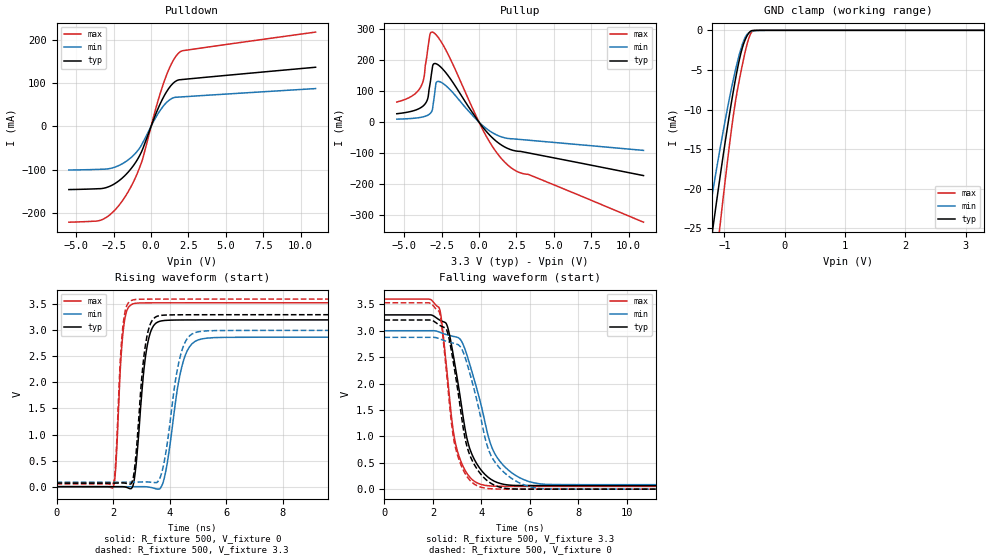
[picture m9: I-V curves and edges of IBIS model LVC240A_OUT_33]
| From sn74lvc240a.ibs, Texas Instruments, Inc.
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[Model]   LVC240A_OUT_33
Model_type  3-state
Enable   Active-Low
Vref =   0
Rref =   500
Cref =   50p
Vmeas =   1.5
| variable   typ   min   max
C_comp   5.30pF   4.90pF   6.71pF
| C_pullup   7.07pF   5.60pF   8.53pF
| C_pulldown   6.30pF   4.97pF   7.29pF
| C_tri-state   5.30pF   4.90pF   6.71pF
[Temperature Range]   40   100   -40
| Ambient temperature   25   85   -40
[Voltage range]   3.3   3   3.6
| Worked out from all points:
|   slope of the pulldown table from 0 to 0.495 V, typ, clamps not added: 11.4 ohm
|   slope of the pullup table from 0 to 0.495 V, typ, clamps not added: 16.4 ohm
|   GND clamp passes 1 mA (typ) near -0.64 V on its own axis
|   rising waveform, R_fixture 500, V_fixture 0: 20-80 % time 314ps typ, 478ps min, 199ps max; typ from 0 V to 3.2 V
|   falling waveform, R_fixture 500, V_fixture 3.3: 20-80 % time 766ps typ, 1.07ns min, 555ps max; typ from 3.3 V to 0.068 V
|   rising waveform, R_fixture 500, V_fixture 3.3: 20-80 % time 302ps typ, 468ps min, 195ps max; typ from 0.068 V to 3.3 V
|   falling waveform, R_fixture 500, V_fixture 0: 20-80 % time 742ps typ, 1.01ns min, 548ps max; typ from 3.2 V to 0 V
[GND Clamp]
| LVC240A_OUT_33
|   Voltage   I(typ)   I(min)   I(max)
-5.5V     -311.6mA   -259.3mA   -396.4mA
-1.31V    -31.75mA   -25.83mA   -41.58mA
-1.265V   -29.16mA   -23.69mA   -38.28mA
-1.18V    -24.37mA   -19.75mA   -32.15mA
-1.095V   -19.72mA   -15.94mA   -26.19mA
-1.055V   -17.59mA   -14.21mA   -23.46mA
-880mV    -8.928mA   -7.206mA   -12.33mA
-760mV    -3.983mA   -3.255mA   -6.545mA
-650mV    -1.084mA   -807.5uA   -2.519mA
-590mV    -295.4uA   -275.9uA   -882.9uA
-535mV    -25.82uA   -102.9uA   -89.75uA
3.3V      62.9pA     44.06nA    -1.767nA
[Pulldown]
| LVC240A_OUT_33
|   Voltage   I(typ)   I(min)   I(max)
-5.5V     -146.4mA   -101.1mA   -221.9mA
-3.68V    -144.6mA   -99.84mA   -219.5mA
-3.245V   -143.7mA   -99.3mA    -215.5mA
-2.51V    -134.3mA   -95.46mA   -197mA
-1.765V   -114.4mA   -83.29mA   -164.4mA
-1.14V    -88.8mA    -65.81mA   -125.6mA
-630mV    -58.01mA   -42.52mA   -82.36mA
385mV     34.5mA     24.73mA    49.95mA
995mV     77.77mA    53.81mA    115.3mA
1.47V     99.56mA    65.75mA    151.8mA
1.91V     107.8mA    67.82mA    171.6mA
11V       136.8mA    87.37mA    218.1mA
[Pullup]
| LVC240A_OUT_33
|   Voltage   I(typ)   I(min)   I(max)
-5.5V     27.15mA    9.676mA    64.84mA
-4.47V    35.52mA    12.08mA    84.48mA
-3.88V    47.09mA    15.63mA    115mA
-3.675V   55mA       17.9mA     145.1mA
-3.43V    75.88mA    22.33mA    234.3mA
-3.27V    125.3mA    27.62mA    284.1mA
-3.065V   185.7mA    57.97mA    288.8mA
-2.875V   188mA      125.7mA    281.3mA
-2.57V    177.9mA    129.2mA    261.6mA
385mV     -24.04mA   -16.62mA   -36.62mA
1.895V    -84.17mA   -52.11mA   -136.8mA
11V       -171.9mA   -90.86mA   -321.9mA
[Ramp]
| LVC240A_OUT_33
| variable   typ   min   max
dV/dt_r   1.94/3.21E-10   1.75/4.88E-10   2.13/2.07E-10
dV/dt_f   1.94/7.70E-10   1.75/1.08E-09   2.13/5.61E-10
R_load = 500
[Rising Waveform]
| LVC240A_OUT_33
R_fixture =   500
C_fixture =   0
L_fixture =   0
V_fixture =   0
V_fixture_min = 0
V_fixture_max = 0
|   Time   V(typ)   V(min)   V(max)
0s        876.5pV    2.928nV    28.8nV
2.005ns   -639.9uV   -125.8uV   -5.276mV
2.095ns   -664.2uV   -275.8uV   381.8mV
2.375ns   -2.243mV   -557.8uV   3.066V
2.805ns   373.8mV    -421.8uV   3.52V
3.22ns    2.74V      -4.637mV   3.527V
3.805ns   3.188V     149.6mV    3.528V
4.49ns    3.199V     2.417V     3.528V
5.31ns    3.2V       2.85V      3.529V
50ns      3.201V     2.87V      3.529V
[Falling Waveform]
| LVC240A_OUT_33
R_fixture =   500
C_fixture =   0
L_fixture =   0
V_fixture =   3.3
V_fixture_min = 3
V_fixture_max = 3.6
|   Time   V(typ)   V(min)   V(max)
0s        3.3V       3V         3.6V
2.245ns   3.211V     2.979V     3.443V
2.6ns     3.077V     2.921V     2.126V
2.81ns    2.613V     2.897V     1.198V
2.99ns    2.128V     2.877V     752.5mV
3.48ns    823.6mV    2.422V     249.1mV
4.18ns    263.9mV    1.196V     70.53mV
4.99ns    86.09mV    411.2mV    52.84mV
6.67ns    68.28mV    90.11mV    52.15mV
50ns      68.11mV    84.91mV    51.97mV
[Rising Waveform]
| LVC240A_OUT_33
R_fixture =   500
C_fixture =   0
L_fixture =   0
V_fixture =   3.3
V_fixture_min = 3
V_fixture_max = 3.6
|   Time   V(typ)   V(min)   V(max)
0s        68.08mV    84.86mV    51.96mV
2ns       68.19mV    84.73mV    53.39mV
2.355ns   70.42mV    84.92mV    3.111V
2.79ns    502.7mV    87.11mV    3.592V
3.075ns   2.422V     91.11mV    3.598V
3.33ns    3.137V     86.06mV    3.599V
3.755ns   3.29V      338.4mV    3.599V
4.455ns   3.298V     2.648V     3.6V
5.12ns    3.299V     2.981V     3.6V
50ns      3.3V       3V         3.6V
[Falling Waveform]
| LVC240A_OUT_33
R_fixture =   500
C_fixture =   0
L_fixture =   0
V_fixture =   0
V_fixture_min = 0
V_fixture_max = 0
|   Time   V(typ)   V(min)   V(max)
0s        3.203V     2.875V     3.53V
2.245ns   3.113V     2.853V     3.369V
2.6ns     2.97V      2.794V     2.011V
2.79ns    2.543V     2.77V      1.156V
2.975ns   2.019V     2.746V     702.8mV
3.425ns   774.4mV    2.348V     225.2mV
4.175ns   185.9mV    923mV      18.34mV
5.065ns   11.71mV    264.3mV    724.3uV
6.65ns    186.1uV    4.311mV    188.2uV
50ns      25.41uV    47.21uV    7.548uV
